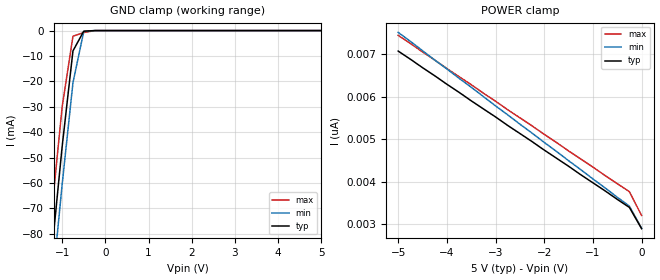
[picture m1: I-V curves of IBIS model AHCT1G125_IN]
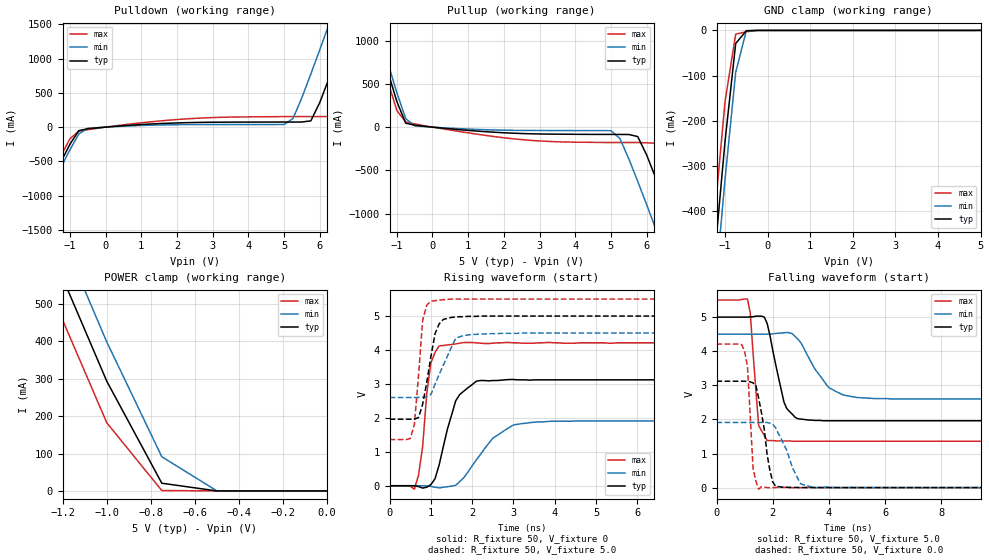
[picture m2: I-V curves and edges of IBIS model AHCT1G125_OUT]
| TEXAS INSTRUMENTS INCORPORATED
| Standard Linear and Logic Group
| IBIS Model of SN74AHCT1G125
| SINGLE BUS BUFFER GATE WITH 3-STATE OUTPUTS
| SOT 5-pin (DCK) and SOT 5-pin (DBV) Package
[IBIS Ver]   3.2
[Comment Char]  |_char
[File Name]   ahct1g125.ibs
[File Rev]   2.0 H_die
[Date]   May 24, 2000
[Source]   Data created from HSPICE simulations at TI-SLL.
[Notes]   The following is an IBIS list for the AHCT1G125.
|   Please contact sllibis@ti.com with questions and
|   comments concerning SLL IBIS models.
[Disclaimer] Property of Texas Instruments Incorporated.  Unauthorized
   reproduction and/or distribution is strictly prohibited.
   This product is protected under copyright law.
   Created 2000, (C) Copyright 2000, Texas Instruments Inc.,
   All Rights Reserved.
   UNLESS THERE IS A SIGNED, WRITTEN AGREEMENT TO THE
   CONTRARY, TEXAS INSTRUMENTS () IS PROVIDING THE IBIS
   MODELS  AND WITHOUT ANY WARRANTY, EXPRESSED OR
   IMPLIED.  TI assumes no liability for:
   1) the accuracy of the IBIS models provided to your
   company;
   2) the proper functioning of these IBIS Models in your
   design or for any resulting applications; or
   3) infringement of patents, copyrights or intellectual
   property rights resulting from your use of these IBIS
   models.
   TI provides IBIS Models as a service to our customers.
   You and your company shall not distribute, sell or give
   these models to anyone else without prior written
   permission from TI.
   TI reserves the right to make changes to our products or
   to discontinue any semiconductor product or service
   without notice, and advises our customers to obtain the
   latest version of relevant information to verify, before
   placing orders, that the information being relied on is
   current.
   Please be aware that your receipt and use of the IBIS
   information provided shall serve as acceptance of these
   terms and conditions.  If you do not accept these terms,
   you should return or destroy the IBIS models and any
   other accompanying information immediately.
|   Component AHCT1G125_DCK
[Component]   AHCT1G125_DCK
[Manufacturer]  Texas Instruments, Inc.
[Package]
|   typ   min   max
R_pkg   0.020   0.017   0.025
L_pkg   0.998nH   0.881nH   1.069nH
C_pkg   0.146pF   0.118pF   0.205pF
[Pin]   signal_name   model_name   R_pin   L_pin   C_pin
1   OE_NOT   AHCT1G125_IN   0.019   1.069nH   0.162pF
2   A   AHCT1G125_IN   0.018   0.881nH   0.121pF
3   GND   GND   0.017   1.031nH   0.205pF
4   Y   AHCT1G125_OUT   0.020   0.960nH   0.124pF
5   VCC   POWER   0.025   1.049nH   0.118pF
|   Component AHCT1G125_DBV
[Component]   AHCT1G125_DBV
[Manufacturer]  Texas Instruments, Inc.
[Package]
|   typ   min   max
R_pkg   0.025   0.021   0.029
L_pkg   1.529nH   1.312nH   1.906nH
C_pkg   0.156pF   0.110pF   0.240pF
[Pin]   signal_name   model_name   R_pin   L_pin   C_pin
1   OE_NOT   AHCT1G125_IN   0.021   1.511nH   0.144pF
2   A   AHCT1G125_IN   0.023   1.312nH   0.138pF
3   GND   GND   0.029   1.906nH   0.240pF
4   Y   AHCT1G125_OUT   0.026   1.541nH   0.150pF
5   VCC   POWER   0.025   1.374nH   0.110pF
| Models and submodels in the file (2): AHCT1G125_IN (Input), AHCT1G125_OUT (3-state)
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|   Model AHCT1G125_IN
[Model]   AHCT1G125_IN
Model_type  Input
Polarity   Inverting
Vinl = 0.8
Vinh = 2.0
| variable   typ   min   max
C_comp   1.16pf   0.87pf   1.45pf
[Temperature Range]   25   85   -40
[Voltage Range]   5.0   4.5   5.5
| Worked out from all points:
|   GND clamp passes 1 mA (typ) near -0.52 V on its own axis
[GND Clamp]
|   Voltage   I(typ)   I(min)   I(max)
-5V       -773mA     -786mA     -758mA
-1.5V     -133mA     -148mA     -117mA
-1.25V    -88.7mA    -104mA     -72.7mA
-1V       -45.6mA    -60.5mA    -30mA
-750mV    -7.99mA    -20.5mA    -2.23mA
-500mV    -233uA     -353uA     -759uA
-250mV    -2.63nA    -182nA     -26.9uA
5V        2.9nA      3.64nA     2.54nA
[POWER Clamp]
|   Voltage   I(typ)   I(min)   I(max)
-5V       7.08nA     7.52nA     7.45nA
-1.5V     4.37nA     4.5nA      4.73nA
-250mV    3.4nA      3.43nA     3.77nA
0V        2.9nA      2.91nA     3.21nA
|   Model AHCT1G125_OUT
[Model]   AHCT1G125_OUT
Model_type  3-state
Polarity   Non-Inverting
Enable   Active-Low
Vmeas = 2.5v
Cref = 15pf
| variable   typ   min   max
C_comp   4.1pf   3.075pf   5.125pf
[Temperature Range]   25   85   -40
[Voltage Range]   5.0   4.5   5.5
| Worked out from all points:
|   slope of the pulldown table from 0 to 0.75 V, typ, clamps not added: 24.8 ohm
|   slope of the pullup table from 0 to 0.75 V, typ, clamps not added: 25.9 ohm
|   GND clamp passes 1 mA (typ) near -0.50 V on its own axis
|   POWER clamp passes 1 mA (typ) near -0.51 V on its own axis
|   rising waveform, R_fixture 50, V_fixture 0: 20-80 % time 398ps typ, 776ps min, 209ps max; typ from 0 V to 3.12 V
|   falling waveform, R_fixture 50, V_fixture 5.0: 20-80 % time 467ps typ, 863ps min, 226ps max; typ from 5 V to 1.96 V
|   rising waveform, R_fixture 50, V_fixture 5.0: 20-80 % time 261ps typ, 415ps min, 161ps max; typ from 1.96 V to 5 V
|   falling waveform, R_fixture 50, V_fixture 0.0: 20-80 % time 345ps typ, 584ps min, 168ps max; typ from 3.12 V to 0 V
[Pulldown]
|   Voltage   I(typ)   I(min)   I(max)
-5V       -4.66A     -4.73A     -4.58A
-2.25V    -1.6A      -1.68A     -1.51A
-2V       -1.32A     -1.4A      -1.23A
-1V       -250mA     -331mA     -170mA
-500mV    -23.5mA    -16.1mA    -37.4mA
5V        74.6mA     38.5mA     154mA
5.75V     91.7mA     776mA      154mA
6.25V     701mA      1.49A      155mA
6.75V     1.42A      2.22A      657mA
7.25V     2.15A      2.96A      1.38A
7.5V      2.52A      3.33A      1.75A
10V       6.23A      7.04A      5.45A
[Pullup]
|   Voltage   I(typ)   I(min)   I(max)
-5V       6.17A      6.26A      6.07A
-1.75V    1.36A      1.46A      1.25A
-1.5V     996mA      1.1A       886mA
-1V       298mA      400mA      194mA
-750mV    45.7mA     98.7mA     59.2mA
-500mV    23mA       14.9mA     37.9mA
5V        -84.3mA    -40.9mA    -178mA
5.75V     -109mA     -626mA     -178mA
6.25V     -581mA     -1.17A     -186mA
6.75V     -1.12A     -1.71A     -574mA
7.25V     -1.67A     -2.27A     -1.12A
10V       -4.73A     -5.33A     -4.18A
[GND Clamp]
|   Voltage   I(typ)   I(min)   I(max)
-5V       -4.66A     -4.73A     -4.58A
-1.5V     -774mA     -858mA     -684mA
-1.25V    -505mA     -590mA     -415mA
-1V       -245mA     -329mA     -157mA
-750mV    -28.8mA    -92.4mA    -8.32mA
-500mV    -878uA     -589uA     -2.99mA
-250mV    -21.8nA    -122nA     -114uA
5V        2nA        199uA      1.9nA
[POWER Clamp]
|   Voltage   I(typ)   I(min)   I(max)
-5V       6.17A      6.26A      6.07A
-1.25V    637mA      743mA      524mA
-1V       293mA      398mA      182mA
-750mV    20.6mA     91.3mA     1.05mA
-500mV    2.09uA     199uA      42uA
0V        2nA        1.97nA     2.2nA
[Ramp]
| variable   typ   min   max
dV/dt_r   1.89E+00/4.25E-10   1.15E+00/7.47E-10   2.52E+00/1.87E-10
dV/dt_f   1.85E+00/4.74E-10   1.17E+00/9.02E-10   2.23E+00/2.48E-10
R_load = 50
[Rising Waveform]
R_fixture = 50
V_fixture = 0
|   Time   V(typ)   V(min)   V(max)
0s        0V         0V         0V
600ps     -498uV     230uV      -101mV
800ps     -68.9mV    -69.3uV    1.16V
1ns       35.6mV     -20mV      3.62V
1.2ns     616mV      -62.9mV    4.12V
1.6ns     2.5V       12.8mV     4.18V
2.2ns     3.1V       923mV      4.2V
3ns       3.13V      1.79V      4.21V
3.9ns     3.12V      1.9V       4.22V
25ns      3.12V      1.91V      4.21V
[Falling Waveform]
R_fixture = 50
V_fixture = 5.0
V_fixture_min = 4.5
V_fixture_max = 5.5
|   Time   V(typ)   V(min)   V(max)
0s        5V         4.5V       5.5V
1.1ns     5V         4.5V       5.53V
1.2ns     5.01V      4.5V       5.13V
1.5ns     5.03V      4.5V       1.82V
1.8ns     4.82V      4.5V       1.38V
2.4ns     2.51V      4.54V      1.37V
2.9ns     2.02V      4.35V      1.36V
4ns       1.96V      2.93V      1.36V
5ns       1.96V      2.64V      1.36V
25ns      1.96V      2.6V       1.36V
[Rising Waveform]
R_fixture = 50
V_fixture = 5.0
V_fixture_min = 4.5
V_fixture_max = 5.5
|   Time   V(typ)   V(min)   V(max)
0s        1.96V      2.6V       1.36V
500ps     1.96V      2.6V       1.39V
600ps     1.96V      2.6V       1.81V
800ps     2.4V       2.61V      4.88V
1ns       3.81V      2.69V      5.44V
1.1ns     4.48V      2.99V      5.45V
1.3ns     4.9V       3.55V      5.48V
1.6ns     4.97V      4.34V      5.5V
2ns       4.99V      4.46V      5.5V
25ns      5V         4.5V       5.5V
[Falling Waveform]
R_fixture = 50
V_fixture = 0.0
|   Time   V(typ)   V(min)   V(max)
0s        3.12V      1.91V      4.21V
1ns       3.12V      1.91V      3.99V
1.1ns     3.11V      1.91V      3.57V
1.3ns     3.07V      1.91V      563mV
1.5ns     2.62V      1.91V      -46.2mV
2ns       170mV      1.86V      -866uV
2.3ns     16.5mV     1.43V      5.8mV
3ns       1.96mV     107mV      -929uV
3.5ns     403uV      -4.39mV    875uV
25ns      0V         0V         0V
